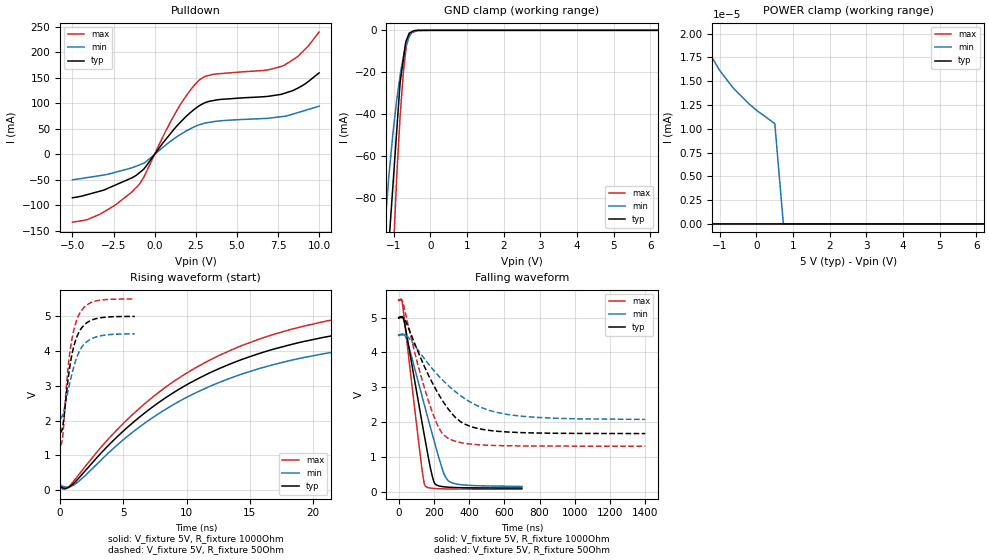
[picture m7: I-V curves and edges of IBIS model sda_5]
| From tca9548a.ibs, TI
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|   sda_5 Model
[Model]   sda_5
Model_type   I/O_open_drain
Polarity   Non-Inverting
Vinl  = 1.5
Vinh  =3.5
Vmeas = 2.5
Vref = 5
Cref = 50pF
Rref = 1000
|   typ   min   max
|   (nom PVT)   (fast PVT)   (slow PVT)
 C_comp   5.695e-12   4.835e-12   6.600e-12
[Model spec]
|subparameter
Vinl   1.5   1.35   1.65
Vinh   3.5   3.15   3.85
| Where nom  PVT is Nominal Process, 5V, 27C
|   Fast PVT is Strong Process,  5.5V, -40C
|   Slow PVT is Weak Process,   4.5V, 125C
[Voltage Range]   5   4.5   5.5
|Junction Temperature
[Temperature Range]   27   125   -40
[Pullup Reference]   5   4.5   5.5
[Pulldown Reference]   0   0   0
[Power Clamp Reference]   5   4.5   5.5
[GND Clamp Reference]   0   0   0
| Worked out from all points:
|   slope of the pulldown table from 0 to 0.75 V, typ, clamps not added: 23.4 ohm
|   GND clamp passes 1 mA (typ) near -0.54 V on its own axis
|   falling waveform, V_fixture 5V, R_fixture 1000Ohm: 20-80 % time 103ns typ, 140ns min, 75.4ns max; typ from 5 V to 0.108 V
|   rising waveform, V_fixture 5V, R_fixture 1000Ohm: 20-80 % time 13.2ns typ, 13.4ns min, 13.2ns max; typ from 0.108 V to 5 V
|   falling waveform, V_fixture 5V, R_fixture 50Ohm: 20-80 % time 203ns typ, 295ns min, 142ns max; typ from 5 V to 1.67 V
|   rising waveform, V_fixture 5V, R_fixture 50Ohm: 20-80 % time 868ps typ, 1.09ns min, 788ps max; typ from 1.67 V to 5 V
[Pulldown]
|   Voltage   I(typ)   I(min)   I(max)
-5V       -85.45mA   -50.22mA   -133.3mA
-3.344V   -72.58mA   -42.04mA   -118.1mA
-2.387V   -60.38mA   -35.36mA   -99.51mA
-946mV    -36.74mA   -21.19mA   -59.33mA
-670mV    -29.56mA   -17.72mA   -45.64mA
610.5mV   26.51mA    16.45mA    41.63mA
1.435V    58.55mA    36.2mA     90.6mA
2.717V    95.16mA    57.84mA    145.7mA
3.785V    106.7mA    64.89mA    157.5mA
7.7V      117.5mA    73.66mA    172.2mA
8.69V     129.3mA    81.54mA    191.4mA
10V       159.5mA    94.28mA    239.6mA
[GND Clamp]
|   Voltage   I(typ)   I(min)   I(max)
-5V       -2.389A    -1.627A    -3.136A
-1.248V   -140.7mA   -95.72mA   -218mA
-1.127V   -101.3mA   -69.04mA   -158mA
-1.022V   -74.58mA   -49.64mA   -111mA
-918.5mV  -48.64mA   -33.63mA   -71.11mA
-825mV    -25.08mA   -21.77mA   -41.4mA
-731.5mV  -13.3mA    -12.48mA   -19.38mA
-670mV    -5.547mA   -7.552mA   -10.14mA
-654.5mV  -4.86mA    -6.696mA   -7.81mA
-566.5mV  -1.255mA   -2.787mA   -1.751mA
-435mV    -80.76uA   -496.4uA   -651.4uA
10V       0A         0A         0A
[POWER Clamp]
|   Voltage   I(typ)   I(min)   I(max)
-5V       618.1uA    634.9uA    852.6uA
-1.793V   443.3nA    406nA      1.386uA
-1.375V   0A         20.82nA    0A
-1.373V   0A         18.52nA    0A
-1.008V   0A         16.15nA    0A
-598.5mV  0A         14.13nA    0A
-202.5mV  0A         12.61nA    0A
-84.44fV  0A         11.95nA    0A
500mV     0A         10.55nA    0A
733.5mV   0A         0A         0A
10V       0A         0A         0A
[Ramp]
R_load = 1000
|   typ   min   max
dV/dt_r   2.93542/1.32326e-08   2.60755/1.33689e-08   3.25425/1.32321e-08
dV/dt_f   2.93536/1.02678e-07   2.60709/1.39566e-07   3.25425/7.54045e-08
[Falling Waveform]
V_fixture = 5V
V_fixture_min = 4.5V
V_fixture_max = 5.5V
R_fixture = 1000Ohm
|   Time   V(typ)   V(min)   V(max)
0s        5V         4.5V       5.5V
21.6ns    5.022V     4.525V     5.398V
51.2ns    4.345V     4.282V     4.122V
131ns     2.039V     2.778V     701.5mV
152.8ns   1.426V     2.364V     150.8mV
178.4ns   727.3mV    1.884V     109.5mV
203.6ns   252.1mV    1.422V     95.26mV
253.8ns   146.7mV    561.3mV    84.7mV
283.6ns   132.7mV    306.9mV    82.08mV
699.8ns   107.7mV    154.8mV    76.25mV
[Rising Waveform]
V_fixture = 5V
V_fixture_min = 4.5V
V_fixture_max = 5.5V
R_fixture = 1000Ohm
|   Time   V(typ)   V(min)   V(max)
0s        107.6mV    154mV      76.23mV
400ps     48.17mV    89.75mV    27.35mV
1.2ns     240.5mV    177.5mV    318.2mV
5ns       1.703V     1.453V     1.922V
9.2ns     2.862V     2.514V     3.184V
13.6ns    3.656V     3.244V     4.048V
19.2ns    4.275V     3.814V     4.715V
26.6ns    4.703V     4.209V     5.179V
33ns      4.873V     4.374V     5.36V
62.8ns    5.001V     4.505V     5.497V
[Falling Waveform]
V_fixture = 5V
V_fixture_min = 4.5V
V_fixture_max = 5.5V
R_fixture = 50Ohm
|   Time   V(typ)   V(min)   V(max)
0s        5V         4.5V       5.5V
23.38ns   4.999V     4.501V     5.437V
53.34ns   4.735V     4.441V     4.801V
114.9ns   3.961V     4.03V      3.539V
191.3ns   3.126V     3.531V     2.278V
237.7ns   2.708V     3.268V     1.752V
283.5ns   2.363V     3.04V      1.529V
403.3ns   1.884V     2.587V     1.373V
617.6ns   1.717V     2.22V      1.321V
1.4us     1.672V     2.077V     1.311V
[Rising Waveform]
V_fixture = 5V
V_fixture_min = 4.5V
V_fixture_max = 5.5V
R_fixture = 50Ohm
|   Time   V(typ)   V(min)   V(max)
0s        1.671V     2.073V     1.311V
120ps     1.709V     2.098V     1.356V
200ps     1.828V     2.17V      1.532V
540ps     2.922V     2.709V     3.195V
800ps     3.643V     3.148V     4.048V
1.12ns    4.196V     3.603V     4.664V
1.52ns    4.569V     3.998V     5.07V
2.06ns    4.805V     4.259V     5.317V
2.92ns    4.944V     4.419V     5.454V
5.9ns     5.001V     4.5V       5.501V
